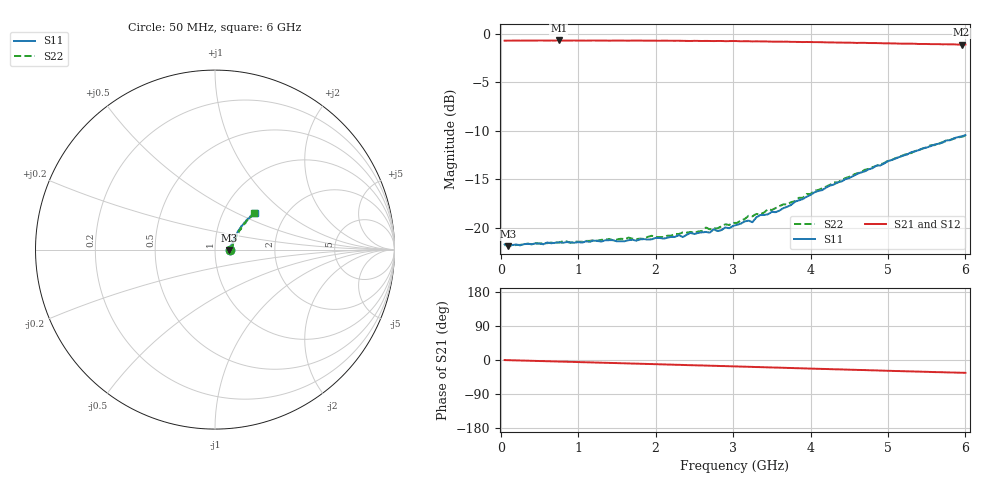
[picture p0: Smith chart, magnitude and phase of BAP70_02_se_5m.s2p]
!	Created	by	janssen	on	Thu	Dec	12	13:21:17	MET	2002
#	HZ	S	MA	R	50
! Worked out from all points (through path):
!   120 points, 50 MHz to 6 GHz, reference 50 ohm
!   highest |S21| = -0.71 dB at 750 MHz (marker M1); lowest = -1.1 dB at 5.95 GHz (marker M2)
!   group delay of S21, straight-line fit = 15.9 ps
!   lowest |S11| = -21.9 dB at 100 MHz (marker M3), VSWR 1.18, Z = 58.8 - j0.17 ohm
!   |S11| at or under -10 dB: start of sweep to end of sweep
!   |S22| runs from -21.8 to -10.5 dB; largest |S21 - S12| = 0.007
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5e7  0.08232 -1.3  0.9194 -0.2  0.9181 -0.3  0.08144 -1.3
1e8  0.08056 -1.0  0.9198 -0.5  0.9193 -0.5  0.0817 -0.9
7.5e8  0.08443 -1.7  0.9216 -4.1  0.9204 -4.1  0.08398 -1.7
1.05e9  0.08402 -1.8  0.9207 -5.8  0.9208 -5.7  0.08489 -2.7
2.05e9  0.08884 4.3  0.9184 -11.3  0.9185 -11.3  0.0896 2.4
2.3e9  0.09182 7.1  0.9185 -12.7  0.9179 -12.7  0.09306 6.8
2.35e9  0.08976 8.1  0.9173 -13.0  0.9179 -13.0  0.0948 7.9
2.45e9  0.09428 9.7  0.9158 -13.7  0.9156 -13.6  0.09538 8.9
2.5e9  0.09313 9.9  0.9174 -13.9  0.9166 -13.9  0.09404 10.0
2.65e9  0.09532 13.4  0.9168 -14.7  0.9164 -14.7  0.1004 11.6
2.7e9  0.09458 14.6  0.9159 -15.0  0.9151 -15.0  0.09831 12.3
2.75e9  0.09836 15.8  0.9149 -15.3  0.9152 -15.3  0.09968 13.0
2.8e9  0.09635 16.3  0.916 -15.6  0.9167 -15.6  0.0995 13.4
3.05e9  0.1038 20.1  0.9148 -17.0  0.9143 -17.0  0.1061 18.1
3.2e9  0.1091 23.0  0.9131 -17.9  0.9132 -17.8  0.1155 21.7
3.25e9  0.107 23.6  0.9112 -18.2  0.9127 -18.1  0.1147 22.1
3.35e9  0.1164 25.3  0.9113 -18.8  0.9113 -18.8  0.1176 24.8
3.6e9  0.1228 30.7  0.9088 -20.2  0.9104 -20.2  0.1296 28.0
4.05e9  0.1523 36.6  0.9037 -23.0  0.9037 -22.7  0.1555 34.8
5.05e9  0.2237 42.7  0.8898 -28.7  0.8942 -28.6  0.2238 40.9
5.95e9  0.2958 42.3  0.8774 -33.6  0.8828 -33.5  0.2941 42.6
6e9  0.3001 42.4  0.8787 -33.9  0.883 -33.9  0.298 42.7
